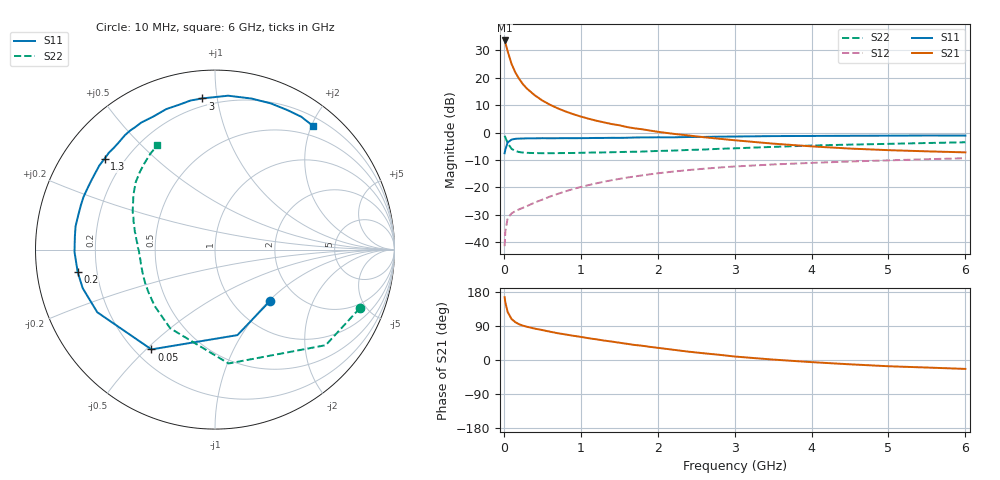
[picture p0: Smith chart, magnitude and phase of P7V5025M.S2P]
! SIEMENS Small Signal Semiconductors
! BFP196
! Si NPN RF Bipolar Junction Transistor in SOT143
! VCE = 0.5 V  IC = 25 mA
! Common Emitter S-Parameters:  May  1996
# GHz  S  MA  R  50
!  f  S11  S21  S12  S22
! GHz  MAG  ANG  MAG  ANG  MAG  ANG  MAG  ANG
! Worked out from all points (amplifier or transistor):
!   36 points, 10 MHz to 6 GHz, reference 50 ohm
!   highest |S21| = 33.5 dB at 10 MHz (marker M1)
!   |S21| within 3 dB of that: start of sweep to 40.73 MHz
!   unconditionally stable (mu >= 1): 513.6 MHz to end of sweep
!   at 250 MHz: K = 0.72, MSG = 22.5 dB, |S12| = -27.4 dB
!   at 1.4 GHz: K = 1.14, MAG = 8.0 dB, |S12| = -17.4 dB
!   at 6 GHz: K = 1.04, MAG = -0.2 dB, |S12| = -9.4 dB
!   S11 on the Smith chart (normalised r, x): 10 MHz: 1.45, -1.02; 50 MHz: 0.26, -0.52; 200 MHz: 0.13, -0.08; 1.3 GHz: 0.13, +0.35; 3 GHz: 0.15, +0.91; 6 GHz: 0.33, +2.02
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0.01  0.4193 -43.4  47.56 165.6  0.0085 75.6  0.8706 -22.0
0.02  0.4925 -75.3  43.18 151.8  0.0159 66.1  0.8149 -40.8
0.05  0.6594 -122.5  30.12 126.6  0.0276 45.0  0.639 -83.2
0.1  0.7431 -152.0  17.84 108.2  0.0336 35.2  0.5043 -119.7
0.15  0.7677 -163.7  12.37 99.7  0.037 34.4  0.4601 -137.0
0.2  0.7752 -170.6  9.439 94.2  0.0399 36.7  0.4403 -147.4
0.25  0.7779 -175.8  7.537 90.5  0.0426 39.2  0.4314 -154.5
0.3  0.7829 -179.1  6.324 87.7  0.0457 41.9  0.4266 -158.8
0.4  0.7842 174.5  4.787 82.9  0.0528 45.8  0.4218 -165.1
0.5  0.7876 170.5  3.832 79.0  0.06 48.6  0.4203 -169.4
0.6  0.7857 165.8  3.205 74.7  0.0681 50.3  0.4196 -172.4
0.7  0.7871 161.7  2.76 70.7  0.0761 51.7  0.4213 -174.8
0.9  0.7882 154.4  2.163 64.1  0.0934 52.3  0.4237 -178.7
1.1  0.7917 147.5  1.788 57.6  0.1101 51.7  0.4305 178.2
1.3  0.7967 140.6  1.531 51.4  0.1268 49.9  0.4343 175.3
1.7  0.8115 128.1  1.192 39.7  0.1582 45.4  0.4468 170.1
2.2  0.8173 114.7  0.949 27.1  0.1943 38.7  0.4683 163.8
3  0.8453 94.8  0.723 9.2  0.2405 27.1  0.5154 152.6
3.5  0.8606 85.1  0.627 1.1  0.2619 20.3  0.5474 146.1
4.5  0.8719 69.1  0.51 -11.4  0.2967 8.6  0.602 134.1
5.5  0.8825 57.0  0.454 -19.9  0.3263 -2.0  0.6438 124.1
6  0.8792 51.6  0.435 -23.5  0.3401 -7.6  0.6639 119.1
